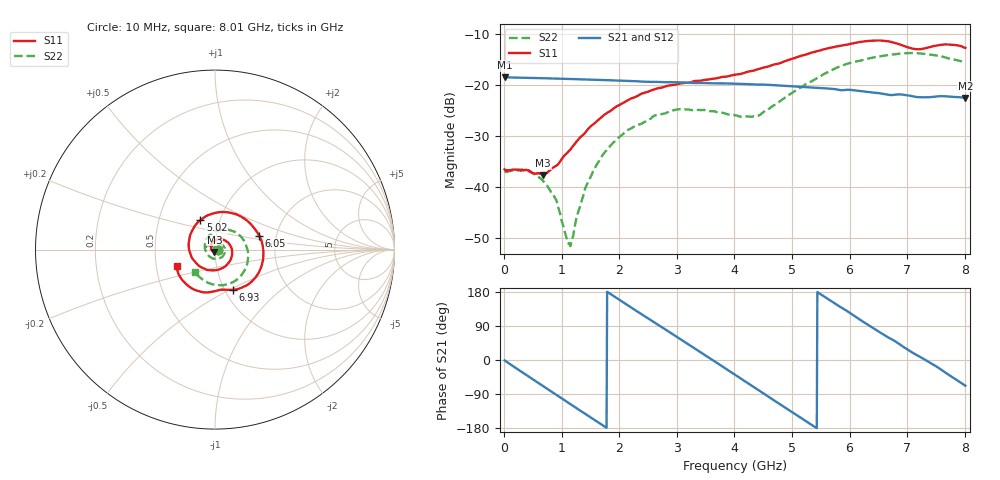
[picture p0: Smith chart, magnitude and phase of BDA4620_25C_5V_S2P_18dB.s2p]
!Agilent Technologies,E5071B,MY42404982,A.09.10
!Date: Wed May 06 09:02:07 2026
!Data & Calibration Information:
!Freq	S11:SOLT2(ON)	S21:SOLT2(ON)	S12:SOLT2(ON)	S22:SOLT2(ON)
# Hz S RI R 50
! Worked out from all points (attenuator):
!   801 points, 10 MHz to 8.01 GHz, reference 50 ohm
!   highest |S21| = -18.42 dB at 10 MHz (marker M1); lowest = -22.5 dB at 8.01 GHz (marker M2)
!   lowest |S11| = -37.7 dB at 680 MHz (marker M3), VSWR 1.03, Z = 49.7 - j1.27 ohm
!   |S11| at or under -10 dB: start of sweep to end of sweep
!   |S22| runs from -51.6 to -13.7 dB; largest |S21 - S12| = 0.00052
!   S11 on the Smith chart (normalised r, x): 10 MHz: 1.03, -0.00; 5.02 GHz: 0.81, +0.27; 6.05 GHz: 1.63, +0.27; 6.93 GHz: 1.09, -0.52; 8.01 GHz: 0.64, -0.13
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1e7  0.0149 -0.00102  0.12 -0.0025  0.1201 -0.0026  0.014 -0.000495
4.2e8  0.00827 -0.0119  0.0865 -0.0804  0.0867 -0.0806  0.0133 -0.00522
6.8e8  -0.00293 -0.0127  0.0419 -0.1095  0.0418 -0.1097  0.00881 -0.00726
8.9e8  -0.0137 -0.00825  -0.000324 -0.1163  -0.00053 -0.1165  0.00336 -0.00692
1.13e9  -0.022 0.00557  -0.0475 -0.1051  -0.0475 -0.1053  -0.00217 -0.00175
1.18e9  -0.0226 0.00934  -0.0563 -0.1003  -0.0565 -0.1005  -0.00292 -3.43e-05
1.35e9  -0.0224 0.0225  -0.0826 -0.0789  -0.0827 -0.079  -0.00471 0.00563
1.58e9  -0.0131 0.0406  -0.1058 -0.0402  -0.1058 -0.0403  -0.00377 0.015
1.87e9  0.0122 0.0559  -0.1106 0.0155  -0.1108 0.0155  0.00445 0.0258
2.16e9  0.046 0.0551  -0.0884 0.066  -0.0885 0.0661  0.0193 0.0311
2.68e9  0.0935 0.00339  -0.00447 0.1077  -0.00433 0.1077  0.0473 0.019
3.07e9  0.0846 -0.0613  0.0627 0.0863  0.063 0.0864  0.0576 -0.00898
4.01e9  -0.0884 -0.0908  0.0806 -0.065  0.0807 -0.0652  -0.0141 -0.0489
4.42e9  -0.1444 0.000459  0.0184 -0.0998  0.0182 -0.1  -0.049 -0.0122
5.02e9  -0.0818 0.1636  -0.0743 -0.0635  -0.0745 -0.0637  -0.0311 0.0798
5.35e9  0.0239 0.2085  -0.094 -0.0131  -0.0941 -0.0131  0.0243 0.1075
6.05e9  0.2462 0.0781  -0.0437 0.0782  -0.0438 0.0783  0.1599 0.0524
6.37e9  0.2665 -0.0626  0.00307 0.085  0.00317 0.0851  0.1843 -0.019
6.68e9  0.1935 -0.1876  0.0418 0.0687  0.0418 0.0689  0.1737 -0.096
6.93e9  0.0992 -0.2241  0.0661 0.0463  0.0664 0.0463  0.1396 -0.1519
7.57e9  -0.0884 -0.2324  0.0716 -0.0313  0.0717 -0.0313  -0.0218 -0.1915
8.01e9  -0.2137 -0.0927  0.0282 -0.0695  0.0283 -0.0696  -0.1101 -0.126
